PROGRAM MAIN
VAR
	bSamplingStart	: BOOL := False;
	nAcuNodeId		: INT := 1;
	iSeq 			: INT;
	nIncCtr			: INT;
	nFirstAcuIndex	: UINT;
	i01Sec:DINT := 0;
	currSync0Count:UINT;
	lastSync0Count:UINT := 0;
	diffSync0:INT := -1;
	
	AcquisitionBlockBuffer			:	 ARRAY [0..nFifoSize] OF stAcquisitionBlock;		(*  Put one Acq Block into fifo buffer *)
	fbBufferAccess	: FB_DataFifo;
		
END_VAR

//IF NOT bSamplingStart THEN
//	ADSLOGSTR(
//				msgCtrlMask := ADSLOG_MSGTYPE_WARN OR ADSLOG_MSGTYPE_LOG,
//				msgFmtStr   := 'SYNC0 not correct %s', 
//				strArg      := '55'
//			);
//END_IF

//IF bSamplingStart THEN
	currSync0Count := AcquisitionData[nAcuNodeId].ECAT_SYNC0_Counter;

	IF diffSync0 < 0 THEN
		lastSync0Count := currSync0Count;
		diffSync0 := 1;
//		ADSLOGSTR(
//				msgCtrlMask := ADSLOG_MSGTYPE_WARN OR ADSLOG_MSGTYPE_MSGBOX,
//				msgFmtStr   := 'Start testing', 
//				strArg      := ''
//			); 
	ELSE
		
		IF diffSync0 <> 1 THEN
			 ADSLOGSTR(
				msgCtrlMask := ADSLOG_MSGTYPE_WARN OR ADSLOG_MSGTYPE_MSGBOX,
				msgFmtStr   := 'SYNC0 not correct %s', 
				strArg      := INT_TO_STRING(diffSync0)
			);      
		END_IF
		
	END_IF

//END_IF


diffSync0 := currSync0Count - lastSync0Count;
lastSync0Count := currSync0Count;


CASE iSeq OF 
0:
	IF bSamplingStart THEN
		iSeq := iSeq + 1;
	END_IF
1:	
	(* reserve for init process *)
	fbBufferAccess.bClearFifo := TRUE;
	IF fbBufferAccess.bFifoEmpty THEN		(* Makesure no data in buffer in inital phase *)
		fbBufferAccess.bClearFifo := FALSE;
		iSeq := 10;
	END_IF
10:	(*  Cyclic Acquisition *)
	nIncCtr := nIncCtr + 1;					(*   Generate a dummy data  *)
	AcquisitionData[nAcuNodeId].ECAT_IRQ_Counter := nIncCtr;
	AcquisitionData[nAcuNodeId].nDcTimeStamp := UInt64Add64( F_GetCurDcTickTime(), EC_DCTIME_DELTA_OFFSET);	(* Shift time from GMT+0 to Current time Zone *)
	
	AcquisitionBlock[nAcuNodeId].DataBlock[nFirstAcuIndex] := AcquisitionData[nAcuNodeId];
	nFirstAcuIndex := nFirstAcuIndex + 1;
	
	IF nFirstAcuIndex > nAcquisitionBlock THEN
		nFirstAcuIndex := 0 ;				(* Block collect finish , put into buffer *)
		fbBufferAccess.bPutData := TRUE;
		
		IF i01Sec < 10 THEN
			i01Sec := i01Sec + 1;
		ELSE
			i01Sec := 0;
			//fbBufferAccess.bFifoFull := FALSE;
		END_IF
		
		IF NOT(bSamplingStart) THEN
			iSeq := 20;			(* Stop Acquisition *)
		END_IF
	END_IF

20:	(* Should call close file process *)
	iSeq := 0;
END_CASE


fbBufferAccess(bPutData:= , 
	bGetData:= , 
	bClearFifo:= , 
	pPutData:= ADR(AcquisitionBlock[nAcuNodeId]), 
	pGetData:= ADR(PRG_DatFileCreat.DatAcqBlock), 
	nDataLen:= SIZEOF(AcquisitionBlock[nAcuNodeId]), 
	pFifoMemory:= ADR(AcquisitionBlockBuffer), 
	nFifoSize:= nFifoSize, 
	bFifoEmpty=> , 
	bFifoFull=> , 
	iFifoSizeLeft=> );


IF fbBufferAccess.bPutData THEN
	fbBufferAccess.bPutData := FALSE;
END_IF; 	
	
IF fbBufferAccess.bGetData THEN
	fbBufferAccess.bGetData := FALSE;
END_IF

PRG_DatFileCreat();

END_PROGRAM
